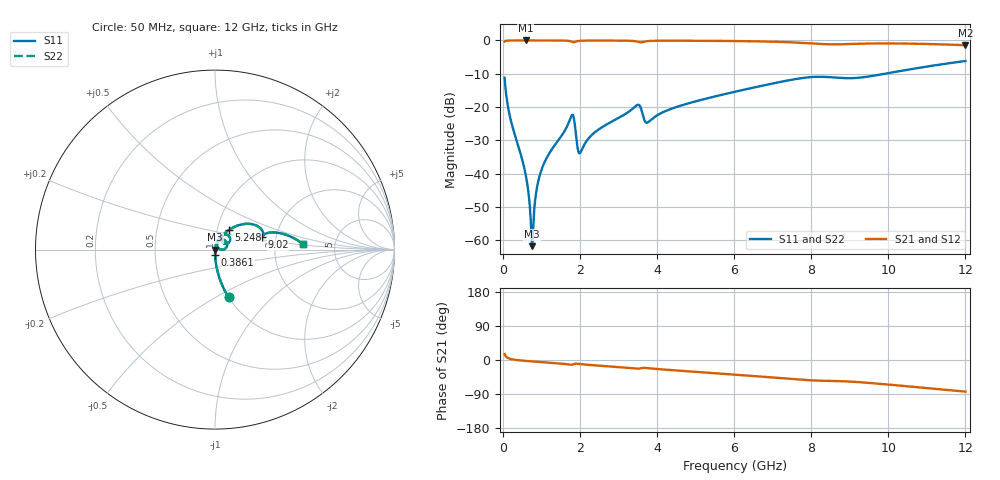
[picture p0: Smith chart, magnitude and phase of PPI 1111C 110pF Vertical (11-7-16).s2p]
# GHz S MA R 50
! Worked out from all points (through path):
!   1601 points, 50 MHz to 12 GHz, reference 50 ohm
!   highest |S21| = -0.01 dB at 602.7 MHz (marker M1); lowest = -1.4 dB at 12 GHz (marker M2)
!   group delay of S21, straight-line fit = 19.1 ps
!   lowest |S11| = -61.8 dB at 759.5 MHz (marker M3), VSWR 1.00, Z = 50.1 - j0.0211 ohm
!   |S11| at or under -10 dB: start of sweep to 9.919 GHz
!   |S22| runs from -61.8 to -6.2 dB; largest |S21 - S12| = 0
!   S11 on the Smith chart (normalised r, x): 50 MHz: 1.00, -0.57; 386.1 MHz: 1.00, -0.06; 5.248 GHz: 1.13, +0.25; 9.02 GHz: 1.68, +0.26; 12 GHz: 2.90, +0.24
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0.05  0.276 -74.2  0.9609 15.8  0.9609 15.8  0.276 -74.2
0.1919063  0.07031 -86.6  0.9971 3.1  0.9971 3.1  0.07031 -86.6
0.3860938  0.02797 -89.1  0.999 -0.3  0.999 -0.3  0.02797 -89.1
0.6026875  0.009185 -88.0  0.9992 -2.4  0.9992 -2.4  0.009185 -88.0
0.7595312  0.0008104 -15.1  0.9992 -3.7  0.9992 -3.7  0.0008104 -15.1
0.8043438  0.002246 64.5  0.9991 -4.1  0.9991 -4.1  0.002246 64.5
0.9014375  0.006728 77.7  0.999 -4.8  0.999 -4.8  0.006728 77.7
1.020938  0.012 79.7  0.9989 -5.7  0.9989 -5.7  0.012 79.7
1.767813  0.06999 53.5  0.9692 -12.4  0.9692 -12.4  0.06999 53.5
1.8425  0.06979 16.8  0.9376 -10.9  0.9376 -10.9  0.06979 16.8
1.969469  0.02083 22.9  0.9824 -10.3  0.9824 -10.3  0.02083 22.9
2.044156  0.02224 53.0  0.99 -11.2  0.99 -11.2  0.02224 53.0
2.395188  0.04191 71.1  0.9955 -14.1  0.9955 -14.1  0.04191 71.1
3.478156  0.1062 50.3  0.9637 -22.8  0.9637 -22.8  0.1062 50.3
3.732094  0.05803 42.3  0.9725 -21.2  0.9725 -21.2  0.05803 42.3
4.038312  0.07695 60.7  0.9897 -24.0  0.9897 -24.0  0.07695 60.7
5.24825  0.1324 55.1  0.9865 -32.9  0.9865 -32.9  0.1324 55.1
6.025  0.1695 49.1  0.9787 -38.7  0.9787 -38.7  0.1695 49.1
8.019156  0.2818 23.7  0.9001 -53.8  0.9001 -53.8  0.2818 23.7
9.019969  0.2705 15.3  0.8838 -57.1  0.8838 -57.1  0.2705 15.3
10.01331  0.3234 17.1  0.902 -64.9  0.902 -64.9  0.3234 17.1
12  0.4907 3.7  0.8475 -83.5  0.8475 -83.5  0.4907 3.7
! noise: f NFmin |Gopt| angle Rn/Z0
0.05  0.0003602  0.862  0.4286  0.0005593
1.372  0.004581  0.7248  6.671  0.003295
2.701  0.008747  0.7195  13.06  0.006095
4.031  0.01647  0.7737  19.47  0.01445
5.36  0.0152  0.6942  25.31  0.009241
6.682  0.02644  0.7754  31.49  0.02231
8.012  0.06758  0.8906  37.66  0.1205
9.341  0.07631  0.8903  43.34  0.1308
10.67  0.05653  0.8406  48.56  0.06252
12  0.05092  0.8111  53.44  0.04498
